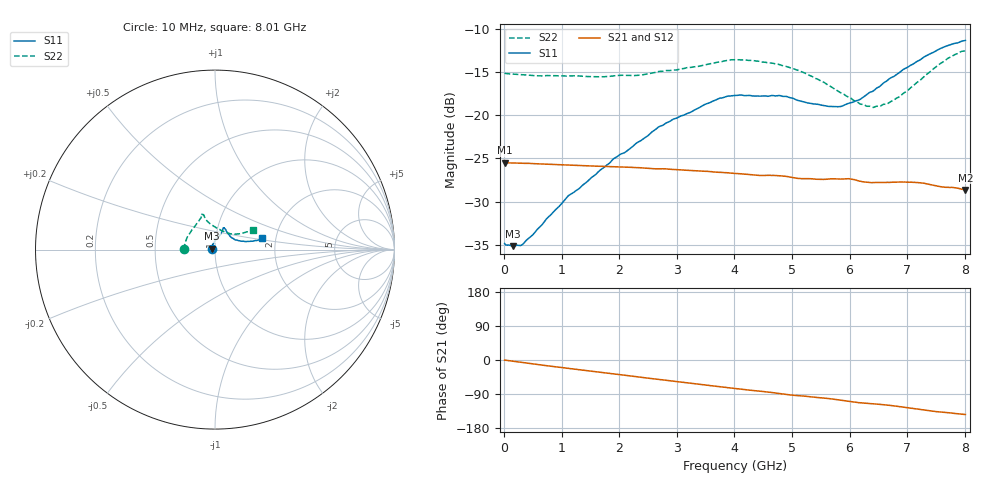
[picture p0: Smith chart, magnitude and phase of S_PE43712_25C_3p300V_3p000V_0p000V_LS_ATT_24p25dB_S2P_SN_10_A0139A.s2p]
! DEVICE ID: PE43712
! File Path: z:\PE43713\PE43713_CHAR_NOM_04292014\AMB\3p300\LS_ATT_24p25dB\PE43713_AMB_3p300V_3p000V_0p000V_LS_ATT_24p25dB_S2P_SN_10_A0139A.s2p
! Serial: 10
! Lot: A0139A
! Temp: 25C
! VDD: 3.300
! VSS: 0.000
! Control_Hi: 3.000
! Control_Lo: 0.000
! Attenuation Step: 24.25dB
! Port 1: RF1
! Port 2: RF2
! ThroughPath:1-2
! IDD: 0.0001450864
! ISS: -6.73e-008
#  Hz  S  RI  R  50
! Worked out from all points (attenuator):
!   801 points, 10 MHz to 8.01 GHz, reference 50 ohm
!   highest |S21| = -25.50 dB at 10 MHz (marker M1); lowest = -28.6 dB at 8.01 GHz (marker M2)
!   lowest |S11| = -35.2 dB at 160 MHz (marker M3), VSWR 1.04, Z = 48.4 + j0.523 ohm
!   |S11| at or under -10 dB: start of sweep to end of sweep
!   |S22| runs from -19.1 to -12.5 dB; largest |S21 - S12| = 0.00019
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1e7  -0.0181 0.000669  0.0531 -0.000232  0.0531 -0.000246  -0.1751 0.00115
1.6e8  -0.0166 0.00541  0.0528 -0.00313  0.0529 -0.00314  -0.1728 0.0114
3.3e8  -0.0151 0.00973  0.0523 -0.00634  0.0523 -0.00628  -0.1704 0.0207
1.1e9  -0.0101 0.0322  0.0478 -0.0191  0.0478 -0.0192  -0.1564 0.0639
1.35e9  -0.00647 0.0384  0.0458 -0.0228  0.0458 -0.0228  -0.1502 0.0757
1.91e9  0.00506 0.056  0.0403 -0.0301  0.0403 -0.0301  -0.1315 0.1068
2.35e9  0.0169 0.0684  0.0351 -0.0352  0.0351 -0.0352  -0.1137 0.1272
2.68e9  0.0272 0.081  0.0309 -0.038  0.0309 -0.038  -0.0999 0.1487
3.71e9  0.0448 0.1157  0.0161 -0.0439  0.0161 -0.0439  -0.0747 0.1885
4.01e9  0.0473 0.1215  0.0118 -0.0445  0.0118 -0.0445  -0.074 0.1965
4.76e9  0.0543 0.1183  0.00147 -0.0446  0.00152 -0.0447  -0.0606 0.188
5.35e9  0.0687 0.0944  -0.00569 -0.0425  -0.00566 -0.0424  -0.0462 0.1612
5.87e9  0.091 0.0671  -0.012 -0.041  -0.0119 -0.041  -0.0109 0.1333
6.17e9  0.1096 0.0559  -0.0161 -0.0384  -0.016 -0.0384  0.0172 0.1156
6.32e9  0.1229 0.0524  -0.0169 -0.0373  -0.0168 -0.0372  0.0346 0.1073
6.51e9  0.1377 0.0486  -0.0184 -0.0365  -0.0184 -0.0364  0.0553 0.0979
6.68e9  0.155 0.0464  -0.0201 -0.0355  -0.02 -0.0355  0.0757 0.0907
6.87e9  0.1716 0.0447  -0.0224 -0.0344  -0.0223 -0.0344  0.0945 0.0869
7.16e9  0.1988 0.046  -0.0258 -0.0316  -0.0257 -0.0316  0.1267 0.0876
7.55e9  0.2357 0.0518  -0.0283 -0.0265  -0.0283 -0.0265  0.171 0.0965
7.81e9  0.2537 0.058  -0.0295 -0.0241  -0.0295 -0.0241  0.1969 0.1058
8.01e9  0.2638 0.0632  -0.0298 -0.0219  -0.0297 -0.0219  0.2094 0.1096
